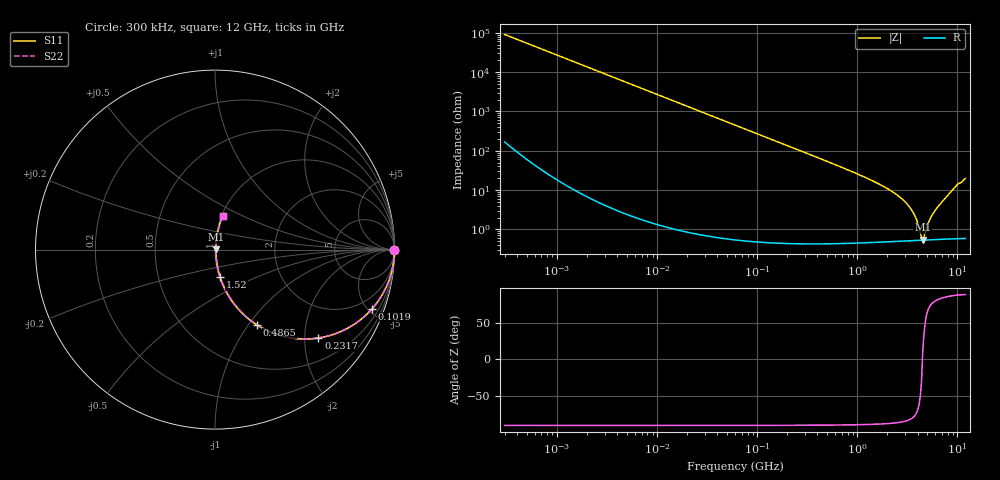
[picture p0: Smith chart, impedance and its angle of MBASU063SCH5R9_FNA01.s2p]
! MBASU063SCH5R9_FNA01  S-PARAMETER MODEL  ( General Type )
! Model Generated by TAIYO YUDEN Corporation (http://www.ty-top.com)
! Version 1.0
! TAIYO YUDEN Control No. 130801
! Copyright(c) 2013 TAIYO YUDEN CO.,LTD. All Rights Reserved.
! Product Description (link to TY-COMPAS)
! https://ds.yuden.co.jp/TYCOMPAS/or/detail?pn=MBASU063SCH5R9DFNA01&u=M
! Products Name : Multilayer Ceramic Capacitors
! Characteristics :
!  Capacitance : 5.9 pF , Rated Voltage : 50V , TCC : CH / C0H
!  Case Size : 0.6 x 0.3 / 0.024 x 0.012 [mm/inch] , Thickness : 0.3 / 0.012 [mm/inch]
!  (Conditions: Temperature = 25 degC , DC Bias Current/Voltage = 0A / 0V)
! External Node Assignments :
!  1  o---| |---o  2
! GND o---------o GND
! Frequency Range : 0.3MHz  -  12000MHz  [ 401 STEP ]
# MHz S RI R 50
! Freq[MHz].  S11 Real  S11 Imag  S21 Real  S21 Imag  S12 Real  S12 Imag  S22 Real  S22 Imag
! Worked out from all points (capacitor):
!   401 points, 300 kHz to 12 GHz, reference 50 ohm
!   read as one part in series: C = 5.87 pF near 316.3 kHz
!   lowest |Z| = 544 mohm at 4.503 GHz (marker M1)
!   series resonance near 4.47 GHz, so ESL is about 220 pH
!   S11 on the Smith chart (normalised r, x): 300 kHz: open; 101.9 MHz: 1.01, -5.32; 231.7 MHz: 1.01, -2.33; 486.5 MHz: 1.01, -1.10; 1.52 GHz: 1.01, -0.32; 12 GHz: 1.01, +0.40
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0.3  1 -0.00111  3.27e-06 0.00111  3.27e-06 0.00111  1 -0.00111
1.769972  1 -0.00653  4.6e-05 0.00653  4.6e-05 0.00653  1 -0.00653
10.44266  0.9985 -0.0385  0.0015 0.0385  0.0015 0.0385  0.9985 -0.0385
27.82928  0.9895 -0.1016  0.0105 0.1016  0.0105 0.1016  0.9895 -0.1016
60  0.953 -0.211  0.047 0.211  0.047 0.211  0.953 -0.211
101.9188  0.8755 -0.3292  0.1245 0.3292  0.1245 0.3292  0.8755 -0.3292
231.6935  0.5761 -0.4923  0.4239 0.4923  0.4239 0.4923  0.5761 -0.4923
353.9943  0.3673 -0.4793  0.6327 0.4793  0.6327 0.4793  0.3673 -0.4793
486.4723  0.2343 -0.4197  0.7657 0.4197  0.7657 0.4197  0.2343 -0.4197
804.7407  0.0992 -0.2923  0.9008 0.2923  0.9008 0.2923  0.0992 -0.2923
1519.776  0.0286 -0.1526  0.9714 0.1526  0.9714 0.1526  0.0286 -0.1526
2088.533  0.0149 -0.0996  0.9851 0.0996  0.9851 0.0996  0.0149 -0.0996
2795.104  0.00845 -0.0585  0.9915 0.0585  0.9915 0.0585  0.00845 -0.0585
3364.605  0.00634 -0.0348  0.9937 0.0348  0.9937 0.0348  0.00634 -0.0348
3740.715  0.00566 -0.0218  0.9943 0.0218  0.9943 0.0218  0.00566 -0.0218
4270.516  0.0053 -0.00582  0.9947 0.00582  0.9947 0.00582  0.0053 -0.00582
4502.883  0.0053 0.00105  0.9947 -0.00105  0.9947 -0.00105  0.0053 0.00105
4747.894  0.00537 0.00602  0.9946 -0.00602  0.9946 -0.00602  0.00537 0.00602
5420.343  0.00579 0.0192  0.9942 -0.0192  0.9942 -0.0192  0.00579 0.0192
6188.031  0.00662 0.0333  0.9934 -0.0333  0.9934 -0.0333  0.00662 0.0333
9708.23  0.0217 0.125  0.9783 -0.125  0.9783 -0.125  0.0217 0.125
12000  0.0431 0.1888  0.9569 -0.1888  0.9569 -0.1888  0.0431 0.1888
